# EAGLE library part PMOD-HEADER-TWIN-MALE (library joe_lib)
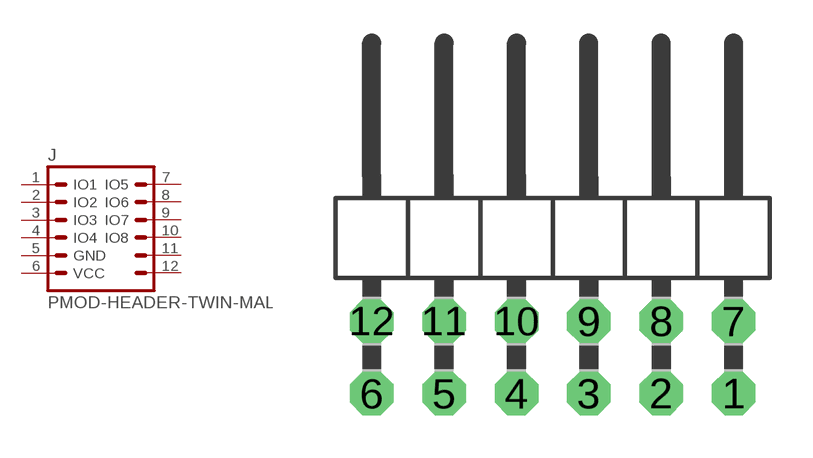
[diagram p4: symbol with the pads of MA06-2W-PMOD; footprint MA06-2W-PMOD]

Designator prefix J

## PMOD-HEADER-TWIN-MALE  [MA06-2W-PMOD]
1  IO1
2  IO2
3  IO3
4  IO4
5  GND  pwr
6  VCC  pwr
7  IO5
8  IO6
9  IO7
10  IO8
11  GND2  pwr
12  VCC2  pwr

## Footprint MA06-2W-PMOD (pad centres in mm)
PMOD Periphal PIN HEADER Pinout from https://reference.digilentinc.com/_media/reference/pmod/pmod-interface-specification-1_2_0.pdf (page 4) Male 6x2 angled header connector
drill 1.016 octagon: 1 5.08,-1.27; 2 2.54,-1.27; 3 0,-1.27; 4 -2.54,-1.27; 5 -5.08,-1.27; 6 -7.62,-1.27; 7 5.08,1.27; 8 2.54,1.27; 9 0,1.27; 10 -2.54,1.27; 11 -5.08,1.27; 12 -7.62,1.27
